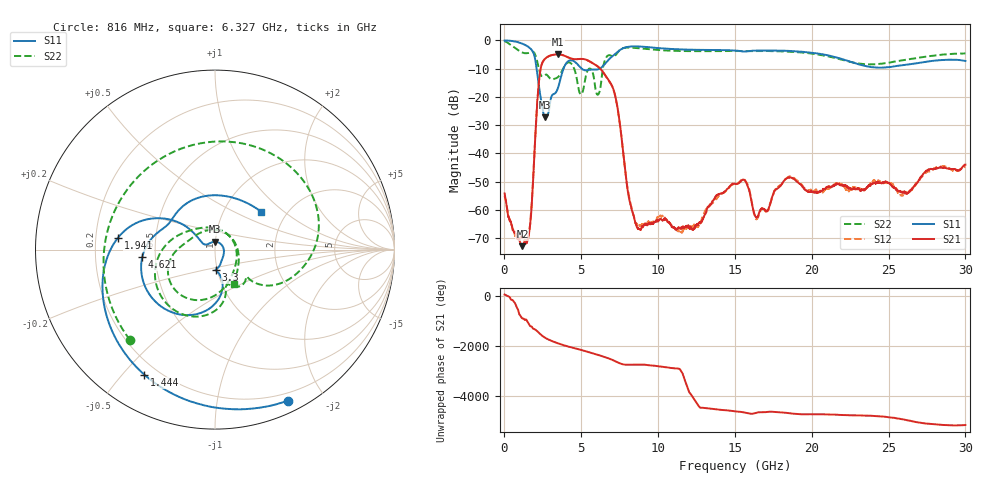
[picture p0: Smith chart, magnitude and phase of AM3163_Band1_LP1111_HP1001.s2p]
!Agilent Technologies,E8364B,MY43040894,A.07.50.67
!Agilent E8364B: A.07.50.67
!Date: Thursday, August 20, 2020 11:59:59
!Correction: S11(Full 2 Port(1,2))
!S21(Full 2 Port(1,2))
!S12(Full 2 Port(1,2))
!S22(Full 2 Port(1,2))
!S2P File: Measurements: S11, S21, S12, S22:
# Hz S  dB  R 50
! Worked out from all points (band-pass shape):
!   3201 points, 10 MHz to 30 GHz, reference 50 ohm
!   highest |S21| = -4.98 dB at 3.468 GHz (marker M1); lowest = -72.8 dB at 1.172 GHz (marker M2)
!   |S21| within 3 dB of the highest: 2.463 GHz to 5.707 GHz (3.244 GHz wide, 79.4 % of centre)
!   lowest |S11| = -27.2 dB at 2.653 GHz (marker M3), VSWR 1.09, Z = 49.6 + j4.31 ohm
!   |S11| at or under -10 dB: 2.09 GHz to 3.845 GHz (1.755 GHz wide, 59.1 % of centre); 5.023 GHz to 6.21 GHz (1.187 GHz wide, 21.1 % of centre)
!   |S22| runs from -19.3 to -0.3 dB; largest |S21 - S12| = 0.0047
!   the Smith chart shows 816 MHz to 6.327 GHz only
!   S11 on the Smith chart (normalised r, x): 816 MHz: 0.12, -1.59; 1.444 GHz: 0.15, -0.57; 1.941 GHz: 0.30, +0.06; 3.3 GHz: 0.98, -0.23; 4.621 GHz: 0.42, -0.04; 6.327 GHz: 1.50, +0.71
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1e7  -0.06 -5.0  -54.20 61.0  -54.97 -41.6  -0.32 -12.0
8.159812e8  -0.59 -64.1  -69.63 -110.8  -69.48 132.0  -3.21 -133.3
1.172112e9  -1.21 -94.1  -72.84 -172.4  -69.56 69.1  -4.35 168.5
1.443897e9  -1.93 -119.4  -71.50 110.4  -71.12 102.4  -4.58 120.8
1.940606e9  -5.28 173.1  -41.10 120.1  -41.25 121.6  -4.43 15.8
2.652869e9  -27.24 93.0  -6.49 128.5  -6.50 128.4  -12.20 -47.7
3.299528e9  -18.72 -87.2  -5.04 -51.8  -5.04 -51.7  -13.55 -72.2
3.468222e9  -17.09 -79.8  -4.98 -89.2  -4.99 -89.2  -13.10 -74.3
3.927444e9  -8.97 -101.3  -5.52 178.3  -5.54 178.5  -8.94 -94.3
4.620962e9  -7.79 -174.0  -6.70 63.3  -6.68 63.4  -11.46 172.6
5.014581e9  -9.96 159.5  -6.59 -1.5  -6.57 -1.6  -19.05 27.3
6.326644e9  -9.55 38.9  -10.61 117.8  -10.67 117.7  -13.09 -60.7
7.498128e9  -3.51 -100.8  -28.97 -170.2  -28.97 -168.9  -3.46 -168.9
8.510291e9  -2.15 179.3  -64.51 133.9  -64.53 68.0  -2.71 129.7
1.000979e10  -2.76 100.6  -63.91 69.3  -62.62 57.6  -3.45 65.7
1.227778e10  -3.36 9.7  -66.85 -108.0  -65.92 -123.7  -3.85 -15.0
1.5005e10  -3.59 -74.0  -50.75 65.8  -50.84 67.2  -3.79 -92.5
1.640141e10  -3.63 -105.4  -62.70 5.6  -63.33 10.6  -3.79 -126.6
2.000958e10  -4.39 162.5  -53.68 -53.9  -52.83 -49.4  -4.70 135.6
2.274617e10  -8.00 59.7  -52.30 -99.5  -51.93 -101.5  -7.93 20.3
2.500479e10  -9.52 -62.9  -50.52 -173.4  -50.55 -169.5  -7.95 -93.2
3e10  -7.32 104.5  -43.99 -124.1  -44.75 -138.2  -4.66 100.9
